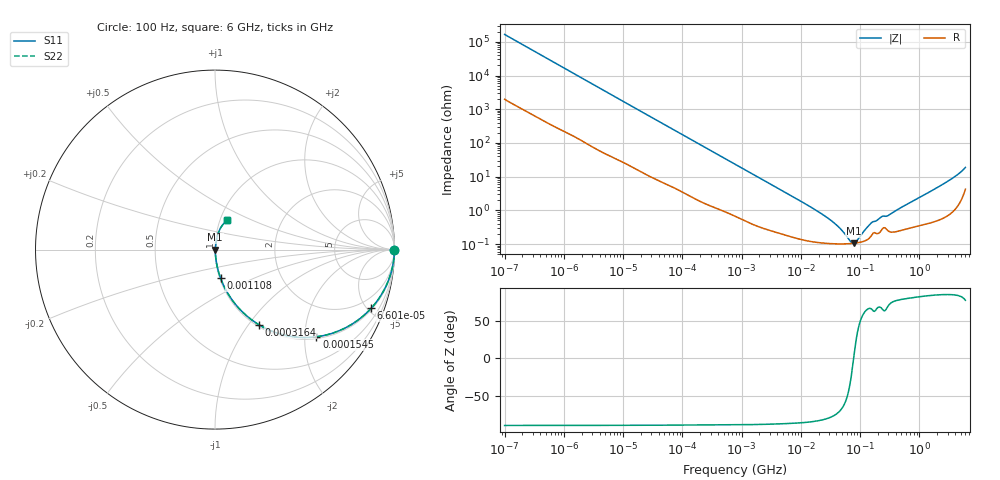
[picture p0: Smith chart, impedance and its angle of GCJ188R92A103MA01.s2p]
!Murata Part Number: GCJ188R92A103MA01
!These Parameters are Measured in Series Mode Connection
!Data Generated on Mar 13, 2026
!  o--ll--o
!Port1  Port2
!  o------o
!Operation Temp=25[degC], DC Bias Voltage=0[V]
!Freq. Start=100[Hz] Stop=6[GHz] 401[Steps]
# Hz S RI R 50
!Freq.(Hz) S11(Real) S11(Imag) S21(Real) S21(Imag) S12(Real) S12(Imag) S22(Real) S22(Imag)
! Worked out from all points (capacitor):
!   401 points, 100 Hz to 6 GHz, reference 50 ohm
!   read as one part in series: C = 9.62 nF near 109 Hz
!   lowest |Z| = 105 mohm at 77.97 MHz (marker M1)
!   series resonance near 77.94 MHz, so ESL is about 430 pH
!   S11 on the Smith chart (normalised r, x): 100 Hz: open; 66 kHz: 1.10, -5.29; 154.5 kHz: 1.05, -2.29; 316.4 kHz: 1.03, -1.13; 1.108 MHz: 1.01, -0.33; 6 GHz: 1.08, +0.36
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100  1 -0.000606  7.6e-06 0.000606  7.6e-06 0.000606  1 -0.000606
2008  0.9997 -0.0119  0.000305 0.0119  0.000305 0.0119  0.9997 -0.0119
12041  0.994 -0.0696  0.00598 0.0696  0.00598 0.0696  0.994 -0.0696
40335  0.9454 -0.2186  0.0546 0.2186  0.0546 0.2186  0.9454 -0.2186
66005  0.8705 -0.3264  0.1295 0.3264  0.1295 0.3264  0.8705 -0.3264
98762  0.7556 -0.42  0.2444 0.42  0.2444 0.42  0.7556 -0.42
154540  0.5652 -0.4858  0.4348 0.4858  0.4348 0.4858  0.5652 -0.4858
316350  0.2456 -0.4191  0.7544 0.4191  0.7544 0.4191  0.2456 -0.4191
774597  0.0572 -0.2183  0.9428 0.2183  0.9428 0.2183  0.0572 -0.2183
1108252  0.0307 -0.1581  0.9693 0.1581  0.9693 0.1581  0.0307 -0.1581
3245845  0.00561 -0.0564  0.9944 0.0564  0.9944 0.0564  0.00561 -0.0564
1.555665e7  0.00131 -0.0117  0.9987 0.0117  0.9987 0.0117  0.00131 -0.0117
3.64232e7  0.00103 -0.00411  0.999 0.00411  0.999 0.00411  0.00103 -0.00411
4.983056e7  0.00101 -0.00228  0.999 0.00228  0.999 0.00228  0.00101 -0.00228
6.817316e7  0.00103 -0.000666  0.999 0.000666  0.999 0.000666  0.00103 -0.000666
7.797396e7  0.00105 2.4e-06  0.9989 -2.4e-06  0.9989 -2.4e-06  0.00105 2.4e-06
8.918374e7  0.00108 0.000675  0.9989 -0.000675  0.9989 -0.000675  0.00108 0.000675
1.526266e8  0.0017 0.00376  0.9983 -0.00376  0.9983 -0.00376  0.0017 0.00376
2.283698e8  0.00255 0.00585  0.9974 -0.00585  0.9974 -0.00585  0.00255 0.00585
3.124326e8  0.00238 0.00696  0.9976 -0.00696  0.9976 -0.00696  0.00238 0.00696
2.142435e9  0.00759 0.0497  0.9924 -0.0497  0.9924 -0.0497  0.00759 0.0497
6e9  0.069 0.1627  0.931 -0.1627  0.931 -0.1627  0.069 0.1627
